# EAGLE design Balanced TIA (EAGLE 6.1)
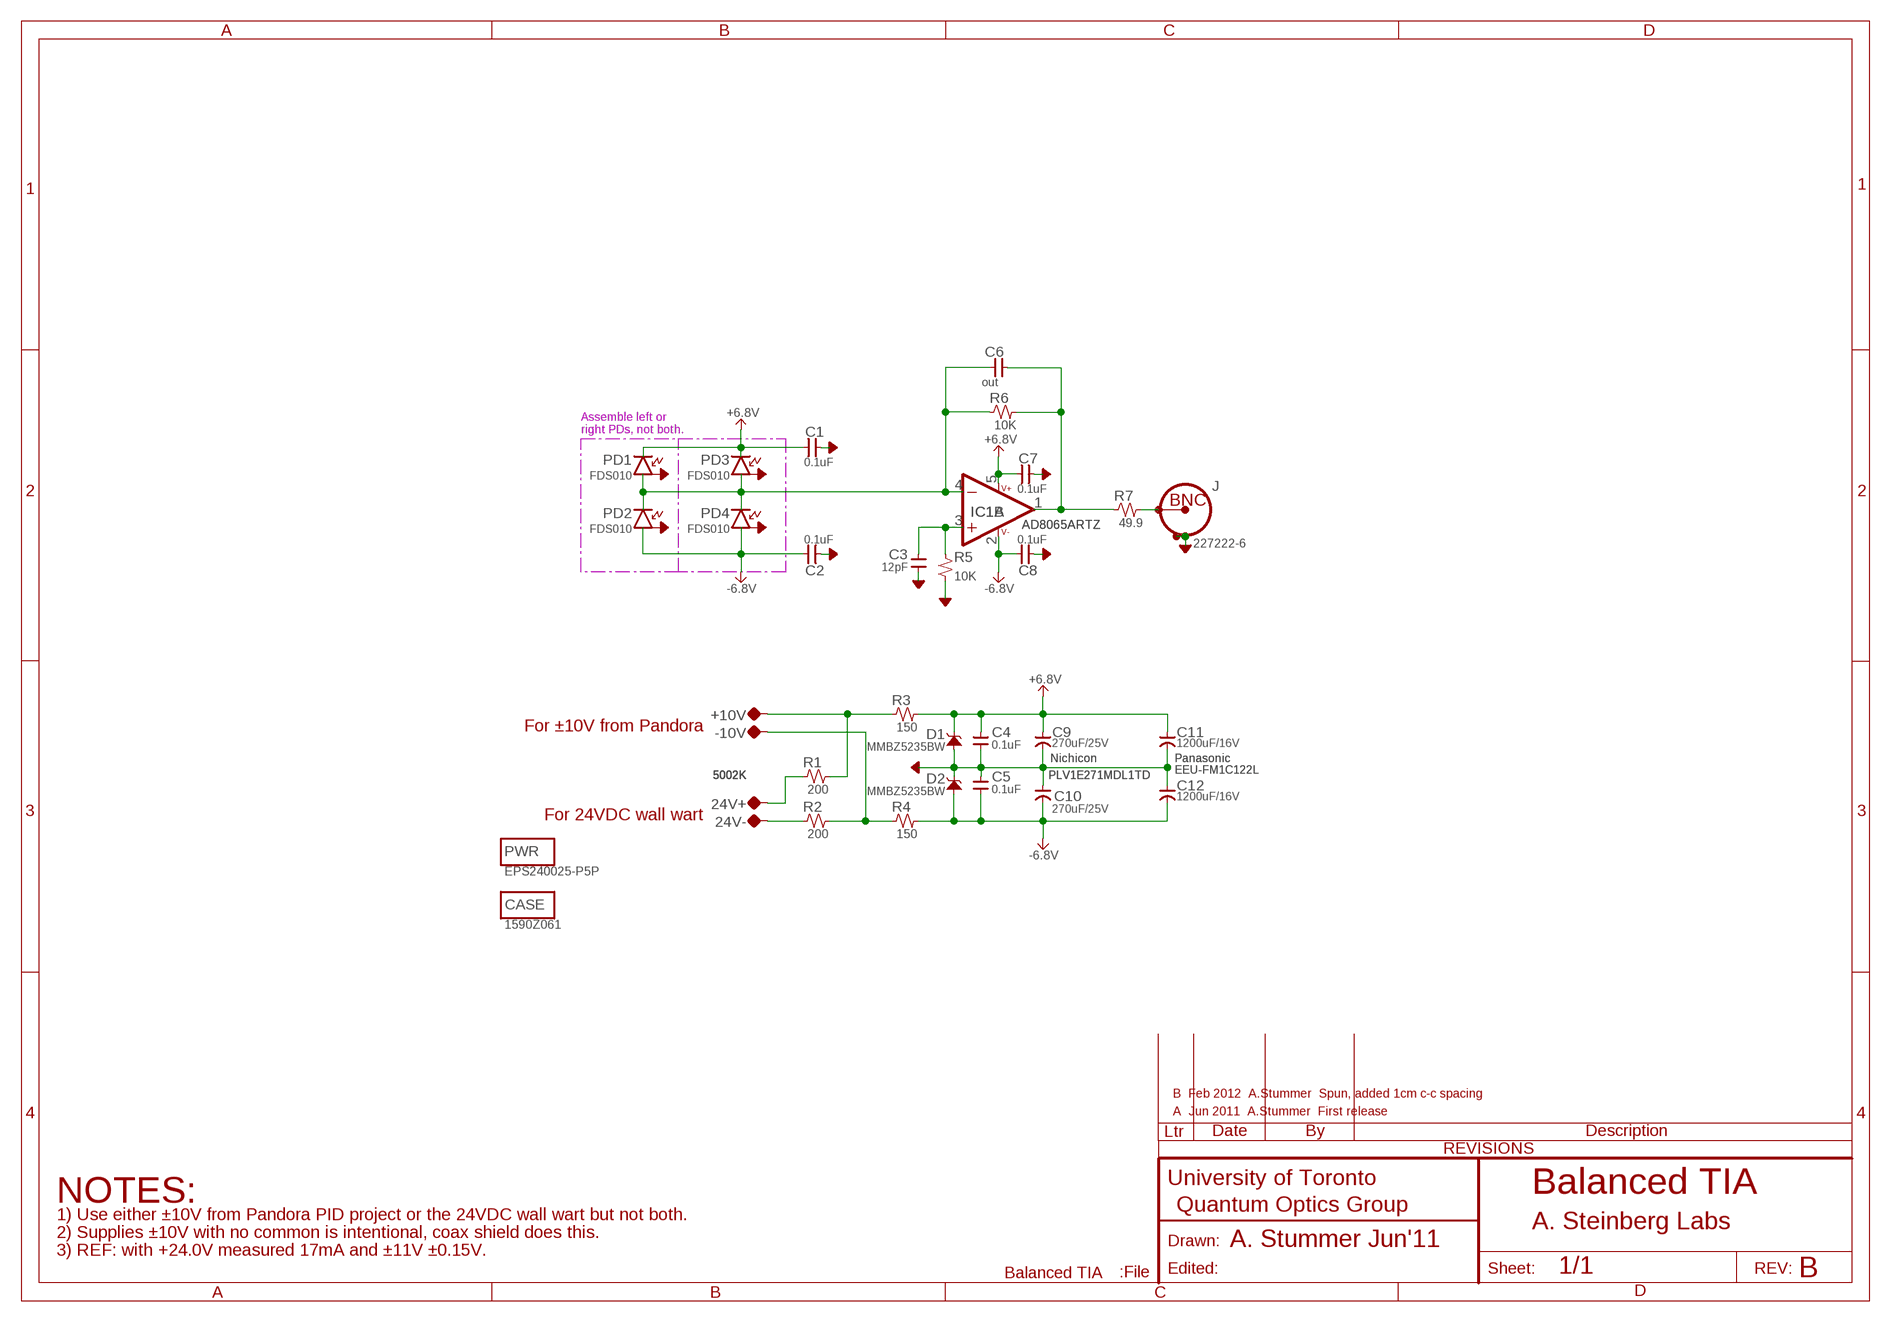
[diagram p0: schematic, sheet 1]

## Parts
24V+  5002K  TP-0.042B  [TP-0.042B]
24V-  5002K  TP-0.042B  [TP-0.042B]
+10V  5002K  TP-0.042B  [TP-0.042B]
-10V  5002K  TP-0.042B  [TP-0.042B]
C1  0.1uF  CAP-H-0805  [2012(0805)]
C2  0.1uF  CAP-H-0805  [2012(0805)]
C3  12pF  CAP-V-0805  [2012(0805)]
C4  0.1uF  CAP-V-0805  [2012(0805)]
C5  0.1uF  CAP-V-0805  [2012(0805)]
C6  out  CAP-H-0805  [2012(0805)]
C7  0.1uF  CAP-H-0805  [2012(0805)]
C8  0.1uF  CAP-H-0805  [2012(0805)]
C9  270uF/25V  CAP-POL--5MM_C-C  [CAP:5MM-THROUGH]
C10  270uF/25V  CAP-POL--5MM_C-C  [CAP:5MM-THROUGH]
C11  1200uF/16V  CAP-POL--5MM_C-C  [CAP:5MM-THROUGH]
C12  1200uF/16V  CAP-POL--5MM_C-C  [CAP:5MM-THROUGH]
CASE  1590Z061  MISC  [MISC]
D1  MMBZ5235BW  ZENER-SOT23  [SOT23]
D2  MMBZ5235BW  ZENER-SOT23  [SOT23]
IC1  AD8065ARTZ  OPAMP-SOT23-5  [SOT23-5]
J  227222-6  CONN:BNC-TYPE2VERT  [CONN:BNC-AMP-TYPE2VERT]
PD1  FDS010  PHOTODIODE:3TERM-FDS010  [PHOTODIODE:3TERM]
PD2  FDS010  PHOTODIODE:3TERM-FDS010  [PHOTODIODE:3TERM]
PD3  FDS010  PHOTODIODE:3TERM-FDS010  [PHOTODIODE:3TERM]
PD4  FDS010  PHOTODIODE:3TERM-FDS010  [PHOTODIODE:3TERM]
PWR  EPS240025-P5P  MISC  [MISC]
R1  200  R-H-0805  [2012(0805)]
R2  200  R-H-0805  [2012(0805)]
R3  150  R-H-0805  [2012(0805)]
R4  150  R-H-0805  [2012(0805)]
R5  10K  R-V-0805  [2012(0805)]
R6  10K  R-H-0805  [2012(0805)]
R7  49.9  R-H-0805  [2012(0805)]

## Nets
+6.8V: C1.1 C4.2 C7.1 C9.+(POS) C11.+(POS) D1.3(C) IC1.5(B:V++) PD1.CATHODE PD3.CATHODE R3.2
-6.8V: C2.1 C5.1 C8.1 C10.-(NEG) C12.-(NEG) D2.1(A) IC1.2(B:V-) PD2.ANODE PD4.ANODE R4.2
AGND: C1.2 C2.2 C3.1 C4.1 C5.2 C7.2 C8.2 C9.-(NEG) C10.+(POS) C11.-(NEG) C12.+(POS) D1.1(A) D2.3(C) J.SHIELD1 J.SHIELD2 PD1.CASE PD2.CASE PD3.CASE PD4.CASE R5.1
N$1 [PD]: C6.1 IC1.4(A:-IN) PD1.ANODE PD2.CATHODE PD3.ANODE PD4.CATHODE R6.1
N$2: C6.2 IC1.1(A:OUT) R6.2 R7.1
N$3: J.CONDUCTOR R7.2
N$4: C3.2 IC1.3(A:+IN) R5.2
N$5: +10V.TP R1.2 R3.1
N$6: -10V.TP R2.2 R4.1
N$7: 24V+.TP R1.1
N$8: 24V-.TP R2.1

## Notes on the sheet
- Assemble left or
- right PDs, not both.
- For ±10V from Pandora
- For 24VDC wall wart
- B  Feb 2012  A.Stummer  Spun, added 1cm c-c spacing
- A  Jun 2011  A.Stummer  First release
- NOTES: | Balanced TIA
- 1) Use either ±10V from Pandora PID project or the 24VDC wall wart but not both.
- A. Steinberg Labs
- 2) Supplies ±10V with no common is intentional, coax shield does this.
- A. Stummer Jun'11
- 3) REF: with +24.0V measured 17mA and ±11V ±0.15V.
- B

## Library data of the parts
24V+ 24V- +10V -10V = QuantumOptics:TP: Testpoint, either SMT pad, small hole or loop style TP such as Keystone 5002K (0.042").
C1 C2 C6-C8 = QuantumOptics:CAP-H-: Cap, SMT and Through-hole, 0402 and up.
C3-C5 = QuantumOptics:CAP-V-: Cap, SMT and Through-hole, 0402 and up.
C9 C10 = QuantumOptics:CAP-POL-: Capacitor, Polarized, SMT 0805 and up, probably tantalum.; MFG: Nichicon; PN: PLV1E271MDL1TD
C11 C12 = QuantumOptics:CAP-POL-: Capacitor, Polarized, SMT 0805 and up, probably tantalum.; MFG: Panasonic; PN: EEU-FM1C122L
CASE PWR = QuantumOptics:MISC: Miscellaneous Part, just a placeholder for miscellaeous parts
D1 D2 = QuantumOptics:ZENER: Zener
IC1 = QuantumOptics:OPAMP: Op Amp, generic, pick the right package. e.g. AD8605: SOT-23-5, RRIO, 10MHz, Ib = 1pA, Vio < 65uV, 2.7-5.5V.
J = QuantumOptics:CONN:BNC: BNC PCB, horizontal or vertical, e.g. Horiz: Amp (5)227677-1, nut 1-329631-2, shoulder washer 330620, vert isolated 5227222-6, http://catalog.tycoelectronics.com/TE/bin/TE.Connect?C=1&M=BYPN&TCPN=5227222-6&RQPN=5227222-6 ...
PD1-PD4 = QuantumOptics:PHOTODIODE:3TERM: Photodiode FDS010, Thorlabs
R1-R4 R6 R7 = QuantumOptics:R-H-*: Resistor, SMT & Through-Hole, horizontal symbol
R5 = QuantumOptics:R-V-*: Resistor, SMT & Through-Hole, vertical symbol

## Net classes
0 default: width 0.178 mm, drill 0.508 mm, clearance 0.178 mm
1 PD: width 0.178 mm, drill 0.508 mm, clearance 0.762 mm

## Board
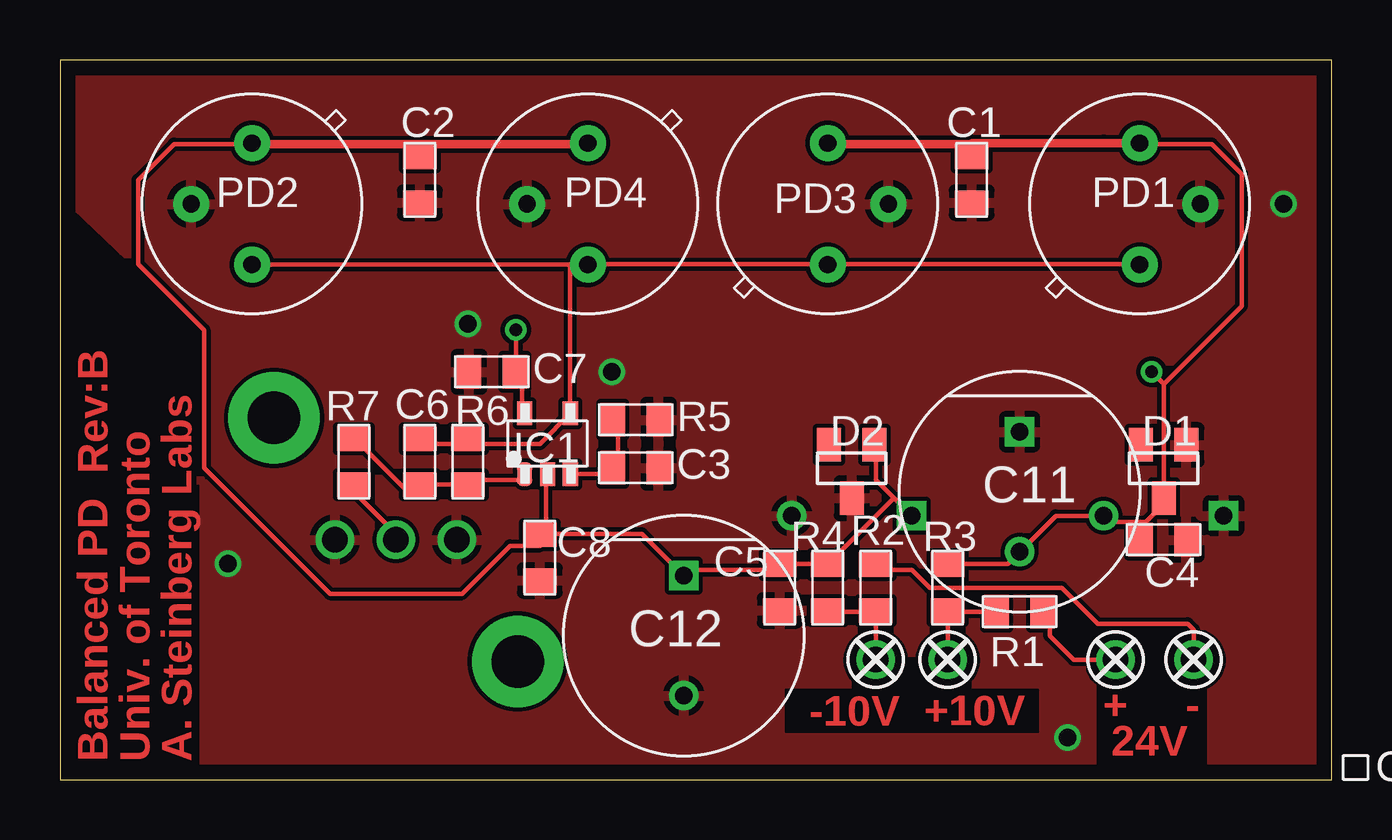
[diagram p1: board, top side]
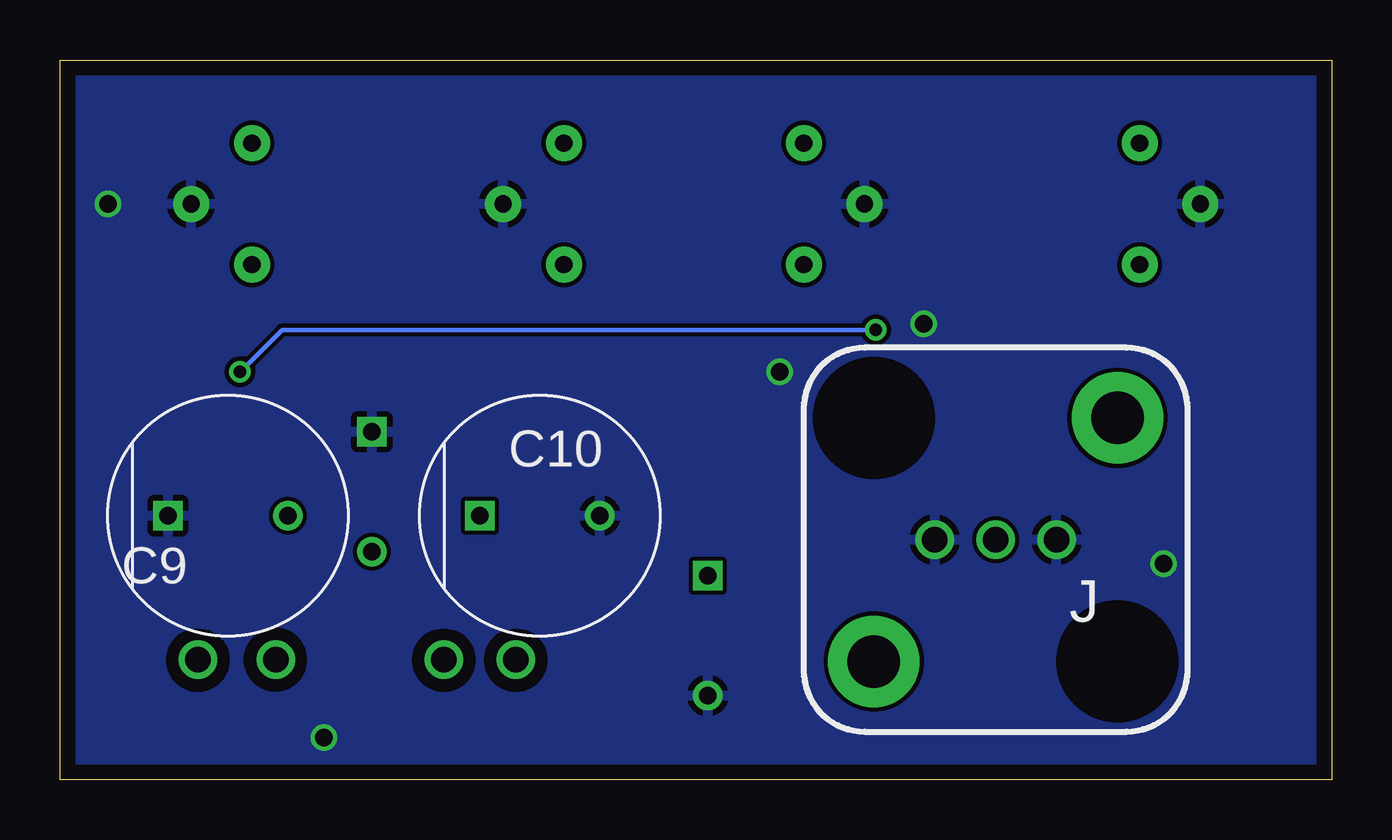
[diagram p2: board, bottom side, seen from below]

Size 53 x 30 mm. Coordinates in mm from the lower left corner, seen from the top.
Outline: 53,0 53,30 0,30 0,0 53,0
Copper layers (1+16): Top 0.035mm / dielectric 1.5mm / Bottom 0.035mm
Design rules: minimum track width 7mil, minimum drill 20mil, track to track 7mil, track to pad 7mil, pad to pad 7mil, via to via 7mil, smd to smd 0mil, copper to edge 25mil, drill to drill 8mil, minimum pad ring 10mil, minimum via ring 8mil, stop-mask expansion 4mil, vias tented up to drill 0mil, thermal gap 10mil
tRestrict: 13 lines
bRestrict: 5 lines

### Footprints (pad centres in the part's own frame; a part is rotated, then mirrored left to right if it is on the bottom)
TP-0.042B = drill 1.067: TP 0,0
2012(0805) = smd 1.016 x 1.397: 1 -0.953,0; 2 0.953,0
CAP:5MM-THROUGH = drill 0.711: + 2.5,0 | drill 0.711 square: - -2.5,0
SOT23 = smd 1 x 1.4: 1 -0.953,-0.953; 2 0.953,-0.953; 3 0,1.27
SOT23-5 = smd 0.635 x 0.991: 1 -0.635,-1.27; 2 0.318,-1.27; 3 1.27,-1.27; 4 1.27,1.27; 5 -0.635,1.27
CONN:BNC-AMP-TYPE2VERT = drill 1.067: CONDUCTOR 0,0; SHIELD1 -2.54,0; SHIELD2 2.54,0 | drill 2.184 pad 3.81: MTG1 -5.08,-5.08; MTG2 5.08,5.08
PHOTODIODE:3TERM = drill 0.711 pad 1.5: ANODE -2.54,0; CASE 0,-2.54; CATHODE 2.54,0

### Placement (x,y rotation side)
24V+  44,5 0 top
24V-  47.25,5 270 top
+10V  37,5 270 top
-10V  34,5 270 top
C1  38,25 270 top
C2  15,25 270 top
C3  24,13 180 top
C4  46,10 180 top
C5  30,8 270 top
C6  15,13.25 270 top
C7  18,17 180 top
C8  20,9.25 270 top
C9  46,11 0 bottom
C10  33,11 0 bottom
C11  40,12 270 top
C12  26,6 270 top
CASE  54,0.5 0 top
D1  46,13 180 top
D2  33,13 180 top
IC1  20,14 0 top
J  14,10 180 bottom
PD1  45,24 90 top
PD2  8,24 270 top
PD3  32,24 90 top
PD4  22,24 270 top
PWR  not placed on the board
R1  40,7 180 top
R2  34,8 270 top
R3  37,8 90 top
R4  32,8 90 top
R5  24,15 180 top
R6  17,13.25 270 top
R7  12.25,13.25 270 top
U$10  [TITLEBLOCK_PCB]  not placed on the board

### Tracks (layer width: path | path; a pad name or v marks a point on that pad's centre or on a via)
+6.8V  (via drill 0.51)
  Top 0.178: 45.25,10.75 45.25,10 C4.2 | 45.25,10.75 46,11.5 D1.3 | 45.25,10.75 43.75,10.75 C9.+ 41.5,11 C11.+ 39.5,9 37,9 R3.2 | 19.25,15.75 19.25,16.75 19,17 | 19.25,15.75 19.25,15.5 IC1.5 19.25,15.75 | 44.75,26.5 45,26.5 PD1.CATHODE | 43.5,26.5 43.5,26.54 | 19,17 v19,18.75 | 19,17 C7.1 | 32,26.5 PD3.CATHODE
  Top 0.18: D1.3 46,16.5 | 46,16.5 49.25,19.75 49.25,25.25 48,26.5 45,26.5 | v45.5,17 46,16.5
  Top 0.36: 44.75,26.5 44.71,26.54 43.5,26.54 38,26.54 38,26.5 | C1.1 38,26.5 | 38,26.5 32,26.5
  Bottom 0.18: v19,18.75 43.75,18.75 v45.5,17
-6.8V
  Top 0.178: 15,26 C2.1 | 32,9 30,9 C5.1 30,8.75 25.75,8.75 | C10.- 34.75,11.75 | 34.75,11.75 34,12.5 34,13.75 D2.1 | 34.75,11.75 32,9 | 32,9 R4.2 | 8,26.5 PD2.ANODE | 6,13 11.25,7.75 16.75,7.75 18.75,9.75 20,9.75 C8.1 | 20.25,10.25 20.25,12.5 IC1.2 | 20.25,10.25 20,10 C8.1 | 20.25,10.25 24.25,10.25 25.75,8.75 | 20.25,10.25 C8.1 | 25.75,8.75 C12.- | 22,26.5 PD4.ANODE
  Top 0.18: 6,13 6,18.75 3.25,21.5 3.25,25 4.75,26.5 8,26.5
  Top 0.36: 8,26.5 15,26.5 | 15,26.5 22,26.5 | 15,26 15,26.5
AGND  (via drill 0.71)
  other vias: 7,9 51,24 23,17 17,19 42,1.75
  pour Bottom (rank 2): 53,0 53,30 0,30 0,0
  pour Top (rank 2): 53,0 53,30 0,30 0,0
N$1
  Top 0.178: R6.1 17,14 15,14 C6.1 | IC1.4 21.25,15.5 21.25,21.46 21.25,21.5 22,21.5 | 22,21.5 32,21.5 | 32,21.5 45,21.5 PD1.ANODE | 32,21.5 PD3.ANODE | 22,21.5 PD4.CATHODE
  Top 0.18: IC1.4 20,14 17.05,14 R6.1 | PD2.CATHODE 21.25,21.46
N$2
  Top 0.178: IC1.1 19.25,12.5 17.25,12.5 17,12.25 R6.2
  Top 0.18: R7.1 12.55,13.95 14.5,12 14.95,12 C6.2 R6.2
N$3
  Top 0.178: 12.25,12 R7.2
  Top 0.18: J.CONDUCTOR 14,10.25 12.25,12
N$4
  Top 0.178: IC1.3 21.5,12.75 22.75,12.75 23,13 C3.2 23.25,13 23.25,15 R5.2
N$5
  Top 0.178: R1.2 37,7 | +10V.TP 37,7 | 37,7 R3.1
N$6
  Top 0.178: 34,7 32,7 R4.1 | -10V.TP 34,7 | 34,7 R2.2
N$7
  Top 0.178: 41,7 R1.1
  Top 0.18: 24V+.TP 42.25,5 41.25,6 41.25,6.75 41,7
N$8
  Top 0.178: 41.75,8 36.25,8 35.5,8.75 34,8.75 R2.1
  Top 0.18: 41.75,8 43.25,6.5 47,6.5 47.25,6.25 24V-.TP

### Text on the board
Top: -10V | + | - | +10V | 24V | Balanced PD Rev:B | Univ. of Toronto | A. Steinberg Labs
Reference: 8 | 37mm | 8 | For outer PDs | OR | 22 | 10mm | 21 | For inner PDs | 6 | 24 | 10 | 26 | Balanced TIA | A. Stummer Jun'11 | B | 0.18mm | 0.5mm | 0.18mm | 0.25mm | 1) The two 1200uF caps placed wherever they fit.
